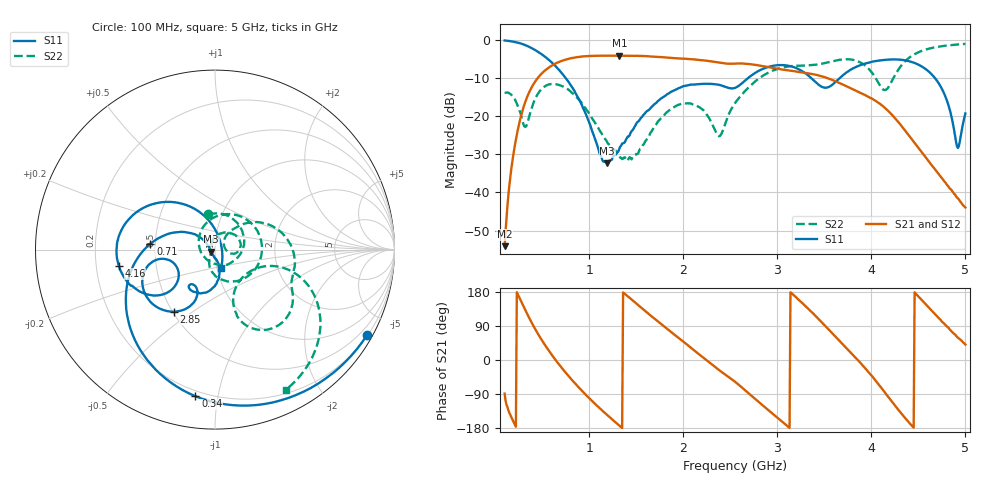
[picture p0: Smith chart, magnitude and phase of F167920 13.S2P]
!  2-Port S-parameters saved by WinCal
! VAR MeasName=S-Parameters (CALIBRATED_DATA) read from VNA (N5242A)
! VAR MeasDate=2016-11-22 9:54:13
! VAR NAME=F167920 13
! VAR FILENAME=F167920 13.S2P
! VAR DATE=2016-11-22 9:54:13
! VAR PHYS_PORTS=1,2
# Hz S DB R 50
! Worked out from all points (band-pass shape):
!   491 points, 100 MHz to 5 GHz, reference 50 ohm
!   highest |S21| = -4.21 dB at 1.32 GHz (marker M1); lowest = -54.0 dB at 100 MHz (marker M2)
!   |S21| within 3 dB of the highest: 576.9 MHz to 2.903 GHz (2.326 GHz wide, 134 % of centre)
!   lowest |S11| = -32.3 dB at 1.19 GHz (marker M3), VSWR 1.05, Z = 47.9 - j1.11 ohm
!   |S11| at or under -10 dB: 747.2 MHz to 2.693 GHz (1.945 GHz wide, 113 % of centre); 3.356 GHz to 3.668 GHz (311.5 MHz wide, 8.87 % of centre); 4.674 GHz to end of sweep
!   |S22| runs from -31.7 to -1.2 dB; largest |S21 - S12| = 0.0017
!   S11 on the Smith chart (normalised r, x): 100 MHz: 0.22, -3.82; 340 MHz: 0.17, -0.86; 710 MHz: 0.47, +0.04; 2.85 GHz: 0.51, -0.42; 4.16 GHz: 0.30, -0.08; 5 GHz: 1.05, -0.22
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1e8  -0.25 -29.3  -54.04 -88.7  -53.42 -91.0  -13.99 100.7
2e8  -0.60 -57.9  -28.97 -165.6  -28.99 -165.8  -15.34 18.0
3.4e8  -1.68 -97.6  -14.99 121.6  -14.98 121.7  -21.92 -170.2
5.1e8  -4.14 -141.4  -8.53 46.8  -8.53 46.8  -12.55 50.7
7.1e8  -8.84 174.8  -5.57 -21.5  -5.57 -21.5  -12.18 -29.1
9.2e8  -17.04 142.5  -4.44 -80.5  -4.44 -80.5  -16.58 -89.1
1.19e9  -32.35 -151.3  -4.22 -144.9  -4.22 -144.9  -26.78 -125.5
1.32e9  -28.54 -99.6  -4.21 -173.0  -4.21 -173.0  -30.40 -141.8
1.5e9  -22.00 -76.6  -4.26 149.3  -4.26 149.3  -29.94 147.1
1.74e9  -15.90 -82.5  -4.57 99.9  -4.56 99.9  -21.18 77.3
2.15e9  -11.70 -113.5  -5.30 18.5  -5.29 18.5  -17.43 -0.9
2.38e9  -11.84 -124.9  -6.04 -26.5  -6.04 -26.5  -25.30 15.9
2.55e9  -12.65 -117.2  -6.30 -57.3  -6.29 -57.3  -16.63 49.0
2.85e9  -7.64 -123.5  -6.97 -120.9  -6.95 -121.0  -9.42 23.6
3.11e9  -6.83 -151.3  -8.05 -175.0  -8.04 -175.2  -7.08 -4.6
3.37e9  -10.30 -170.3  -9.02 125.3  -9.01 125.2  -6.69 -23.1
3.74e9  -8.54 -138.7  -12.28 30.2  -12.26 30.1  -5.16 -47.2
4.16e9  -5.29 -170.5  -18.23 -90.9  -18.23 -91.2  -13.07 -37.1
4.19e9  -5.24 -173.2  -18.94 -100.6  -18.95 -101.0  -12.12 -25.9
4.67e9  -9.89 126.5  -33.72 122.6  -33.79 122.7  -2.07 -44.4
4.92e9  -28.35 9.5  -41.55 59.0  -41.67 59.7  -1.29 -59.4
5e9  -19.34 -71.0  -43.94 40.8  -43.98 41.0  -1.15 -63.3
